(* Logix 5000 AddOnInstructionDefinition export AMCI_3204_AOP_Absolute_Move; software revision 20.03 *)

ADD_ON_INSTRUCTION AMCI_3204_AOP_Absolute_Move   (* revision 1.0, vendor AMCI, ExecuteEnableInFalse *)
VAR_INPUT
   axis_status_bits : INT; {required}
   channel_number : INT; {required}
   _0_normal_1_S_Curve_Acceleration : BOOL;
   _0_Triangular_1_Trapezoidal_S_Curve : BOOL;
   Target_Position : DINT; {required}
   Programmed_speed : DINT; {required}
   Acceleration : DINT; {required}
   Deceleration : DINT; {required}
END_VAR
VAR_IN_OUT
   AMCI_3204_output_data : AM:1756_3204:O:0; {required}
END_VAR
VAR_OUTPUT
   EN : BOOL; {access Read Only, visible}
   ER : BOOL; {access Read Only, visible}
END_VAR
VAR
   command_data_block : DINT[8]; {access None}
END_VAR

ROUTINE EnableInFalse   (* ladder *)
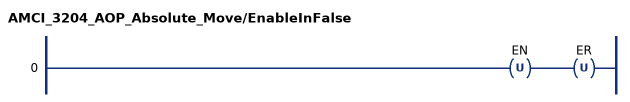
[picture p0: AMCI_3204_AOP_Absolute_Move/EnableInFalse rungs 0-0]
   0: OTU(EN)OTU(ER);
END_ROUTINE

ROUTINE Logic   (* ladder *)
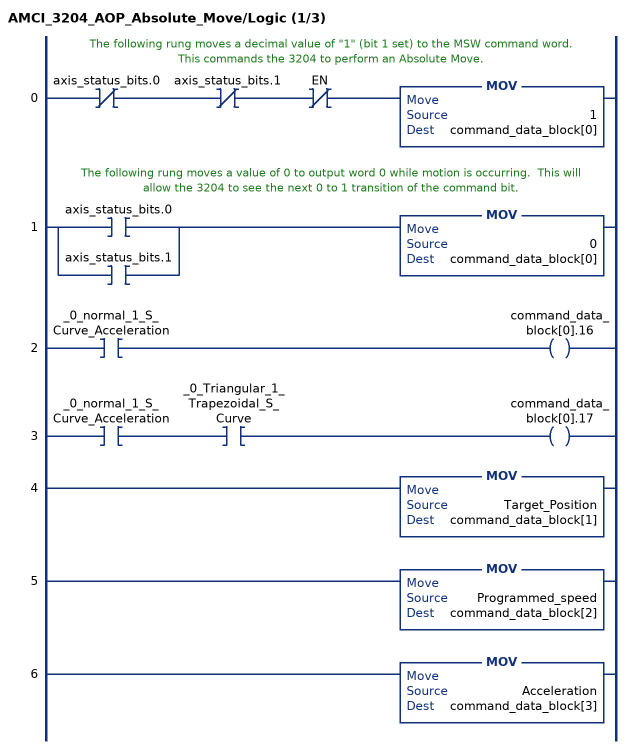
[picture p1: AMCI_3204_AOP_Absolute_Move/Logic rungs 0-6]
   // The following rung moves a decimal value of "1" (bit 1 set) to the MSW command word.  This commands the 3204 to perform an Absolute Move.
   0: XIO(axis_status_bits.0)XIO(axis_status_bits.1)XIO(EN)MOV(1,command_data_block[0]);
   // The following rung moves a value of 0 to output word 0 while motion is occurring.  This will allow the 3204 to see the next 0 to 1 transition of the command bit.
   1: [XIC(axis_status_bits.0) ,XIC(axis_status_bits.1) ]MOV(0,command_data_block[0]);
   2: XIC(_0_normal_1_S_Curve_Acceleration)OTE(command_data_block[0].16);
   3: XIC(_0_normal_1_S_Curve_Acceleration)XIC(_0_Triangular_1_Trapezoidal_S_Curve)OTE(command_data_block[0].17);
   4: MOV(Target_Position,command_data_block[1]);
   5: MOV(Programmed_speed,command_data_block[2]);
   6: MOV(Acceleration,command_data_block[3]);
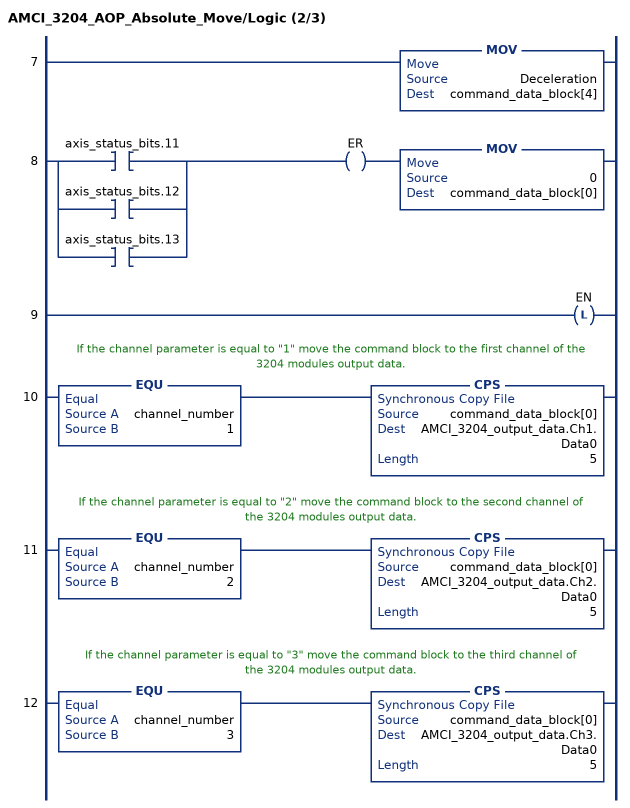
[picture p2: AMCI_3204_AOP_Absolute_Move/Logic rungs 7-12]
   7: MOV(Deceleration,command_data_block[4]);
   8: [XIC(axis_status_bits.11) ,XIC(axis_status_bits.12) ,XIC(axis_status_bits.13) ]OTE(ER)MOV(0,command_data_block[0]);
   9: OTL(EN);
   // If the channel parameter is equal to "1" move the command block to the first channel of the 3204 modules output data.
   10: EQU(channel_number,1)CPS(command_data_block[0],AMCI_3204_output_data.Ch1.Data0,5);
   // If the channel parameter is equal to "2" move the command block to the second channel of the 3204 modules output data.
   11: EQU(channel_number,2)CPS(command_data_block[0],AMCI_3204_output_data.Ch2.Data0,5);
   // If the channel parameter is equal to "3" move the command block to the third channel of the 3204 modules output data.
   12: EQU(channel_number,3)CPS(command_data_block[0],AMCI_3204_output_data.Ch3.Data0,5);
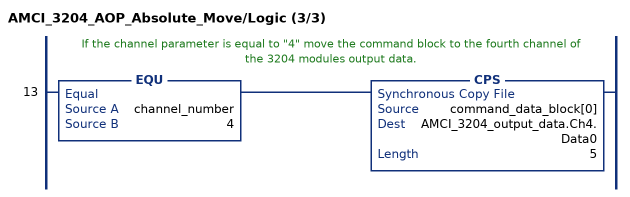
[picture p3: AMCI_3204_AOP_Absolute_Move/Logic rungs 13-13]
   // If the channel parameter is equal to "4" move the command block to the fourth channel of the 3204 modules output data.
   13: EQU(channel_number,4)CPS(command_data_block[0],AMCI_3204_output_data.Ch4.Data0,5);
END_ROUTINE
END_ADD_ON_INSTRUCTION
